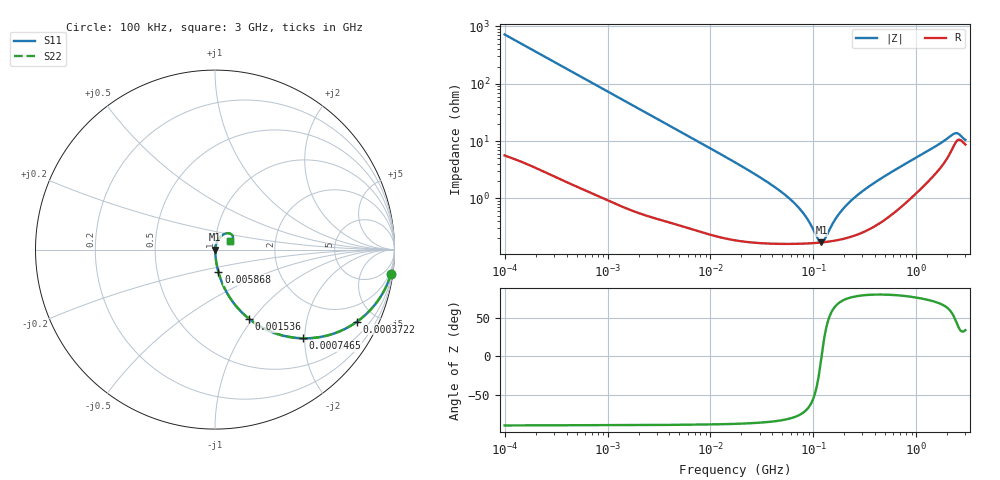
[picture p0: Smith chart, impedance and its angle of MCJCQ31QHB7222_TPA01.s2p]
! MCJCQ31QHB7222_TPA01  S-PARAMETER MODEL  ( Standard Model )
! Model Generated by TAIYO YUDEN Corporation (http://www.ty-top.com)
! Version 1.0
! TAIYO YUDEN Control No. 220601
! Copyright(c) 2015 TAIYO YUDEN CO.,LTD. All Rights Reserved.
! Product Description (link to TY-COMPAS)
! https://ds.yuden.co.jp/TYCOMPAS/or/detail?pn=MCJCQ31QHB7222KTPA01&u=M
! Products Name : Multilayer Ceramic Capacitors
! Characteristics :
!  Capacitance : 2200 [pF] , Rated Voltage : 250 [V] , TCC : X7R
!  Case Size : 3.2 x 1.6 / 0.126 x 0.063 [mm/inch] , Thickness : 1.15 / 0.045 [mm/inch]
!  (Conditions: Temperature = 25 [degC] , DC Bias Voltage = 0 [V])
! External Node Assignments :
!  1  o---| |---o  2
! GND o---------o GND
! Frequency Range : 100kHz  -  3GHz  [ 401 STEP ]
# MHZ S RI R 50
! Freq[MHz].  S11 Real  S11 Imag  S21 Real  S21 Imag  S12 Real  S12 Imag  S22 Real  S22 Imag
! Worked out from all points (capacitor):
!   401 points, 100 kHz to 3 GHz, reference 50 ohm
!   read as one part in series: C = 2.19 nF near 105.3 kHz
!   lowest |Z| = 170 mohm at 119.7 MHz (marker M1)
!   series resonance near 120.1 MHz, so ESL is about 800 pH
!   S11 on the Smith chart (normalised r, x): 100 kHz: 1, -15; 372.2 kHz: 1.04, -3.93; 746.5 kHz: 1.02, -1.97; 1.536 MHz: 1.01, -0.96; 5.868 MHz: 1.01, -0.25; 3 GHz: 1.17, +0.12
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0.1  0.9803 -0.135  0.0197 0.135  0.0197 0.135  0.9803 -0.135
0.21115  0.9204 -0.266  0.0796 0.266  0.0796 0.266  0.9204 -0.266
0.372249  0.7916 -0.401  0.2084 0.401  0.2084 0.401  0.7916 -0.401
0.562235  0.6281 -0.4777  0.3719 0.4777  0.3719 0.4777  0.6281 -0.4777
0.746515  0.4919 -0.494  0.5081 0.494  0.5081 0.494  0.4919 -0.494
1.536162  0.1908 -0.3861  0.8092 0.3861  0.8092 0.3861  0.1908 -0.3861
3.161081  0.0557 -0.2204  0.9443 0.2204  0.9443 0.2204  0.0557 -0.2204
5.867632  0.0188 -0.1241  0.9812 0.1241  0.9812 0.1241  0.0188 -0.1241
17.7727  0.00354 -0.0412  0.9965 0.0412  0.9965 0.0412  0.00354 -0.0412
56.67997  0.00171 -0.0103  0.9983 0.0103  0.9983 0.0103  0.00171 -0.0103
77.22239  0.00165 -0.00571  0.9983 0.00571  0.9983 0.00571  0.00165 -0.00571
97.38194  0.00166 -0.00265  0.9983 0.00265  0.9983 0.00265  0.00166 -0.00265
110.7752  0.00168 -0.00102  0.9983 0.00102  0.9983 0.00102  0.00168 -0.00102
119.6798  0.0017 -4.84e-05  0.9983 4.84e-05  0.9983 4.84e-05  0.0017 -4.84e-05
129.3002  0.00173 0.00092  0.9983 -0.00092  0.9983 -0.00092  0.00173 0.00092
171.6802  0.00189 0.00456  0.9981 -0.00456  0.9981 -0.00456  0.00189 0.00456
216.4987  0.00212 0.00779  0.9979 -0.00779  0.9979 -0.00779  0.00212 0.00779
318.6746  0.00286 0.0142  0.9971 -0.0142  0.9971 -0.0142  0.00286 0.0142
547.5153  0.00553 0.0267  0.9945 -0.0267  0.9945 -0.0267  0.00553 0.0267
2259.438  0.0794 0.0908  0.9206 -0.0908  0.9206 -0.0908  0.0794 0.0908
2504.792  0.0993 0.074  0.9007 -0.074  0.9007 -0.074  0.0993 0.074
3000  0.0827 0.0495  0.9173 -0.0495  0.9173 -0.0495  0.0827 0.0495
